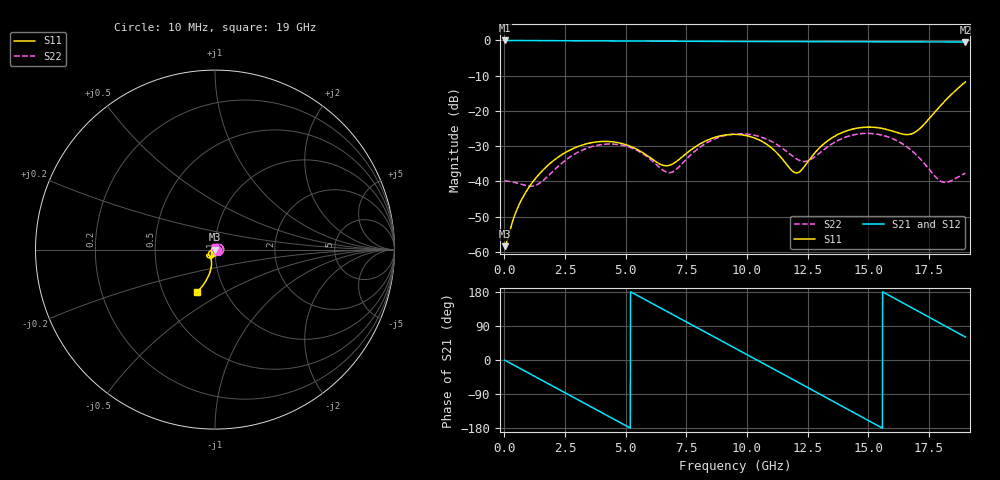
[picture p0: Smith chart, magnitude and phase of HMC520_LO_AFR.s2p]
! Analog Devices, Inc.
! 1 Analog Way
! Wilmington, MA 01887
! http://www.analog.com
! Date:  2021-09-07 NN
! Board Name:  EV1HMC520ALC4 Revision A with HMC520ALC4 installed
! File Description:  Automatic Fixture Removal S-Parameters for LO Port connector and board loss de-embedding
! File Generation:  Calibrated Network Analyzer
! Chip Part Number:  HMC520A
! Chip Description:  GaAs, MMIC, IQ Mixer
! Chip Frequency:  6 to 10 GHz
! Chip Package:  LCC, 3.9 x 3.9 x 0.9 mm
! LO Port:  HMC520ALC4 removed and end of trace left open
!Note:
!  Analog Devices supplies this data as a sample of measured data at the evaluation board
!  ports for this product.  Your particular data for this product may vary.
!  Analog Devices reserves the right to change this data at anytime.
!  All lines below in this file are as is from the Network Analyzer.
!Agilent Technologies,N5245A,MY52451809,A.10.47.06
!Automatic Fixture Removal (AFR)
!Date: Friday, August 27, 2021 11:21:52 PM
!S2P File: Measurements: S11,S21,S12,S22:
# MHz S  RI  R 50
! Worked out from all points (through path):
!   1900 points, 10 MHz to 19 GHz, reference 50 ohm
!   highest |S21| = 0.00 dB at 10 MHz (marker M1); lowest = -0.4 dB at 19 GHz (marker M2)
!   group delay of S21, straight-line fit = 96.3 ps
!   lowest |S11| = -58.4 dB at 10 MHz (marker M3), VSWR 1.00, Z = 50.1 + j0.0055 ohm
!   |S11| at or under -10 dB: start of sweep to end of sweep
!   |S22| runs from -41.4 to -26.4 dB; largest |S21 - S12| = 1.4e-15
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10  0.0012 5.49e-05  0.9999 -0.00602  0.9999 -0.00602  0.0101 2.59e-06
580  0.0037 0.00247  0.9371 -0.3413  0.9371 -0.3413  0.00931 0.000527
1200  0.0101 0.00102  0.7453 -0.6575  0.7453 -0.6575  0.008 0.00317
2210  0.0173 -0.0135  0.2332 -0.9608  0.2332 -0.9608  0.0119 0.0111
3180  0.00897 -0.0312  -0.3365 -0.9254  -0.3365 -0.9254  0.025 0.0114
4820  -0.0193 -0.0287  -0.9526 -0.2225  -0.9526 -0.2225  0.0278 -0.0172
5570  -0.0203 -0.0181  -0.9516 0.2167  -0.9516 0.2167  0.0108 -0.0239
6340  -0.0124 -0.0132  -0.7521 0.619  -0.7521 0.619  -0.0077 -0.0144
6920  -0.00574 -0.0166  -0.4938 0.8381  -0.4938 0.8381  -0.0135 0.00176
7900  -0.00496 -0.031  0.0561 0.9691  0.0561 0.9691  0.00212 0.0276
8670  -0.0161 -0.0389  0.4828 0.8403  0.4828 0.8403  0.0279 0.0286
9510  -0.031 -0.0345  0.8285 0.5  0.8285 0.5  0.0466 0.00599
10990  -0.0288 -0.00907  0.9067 -0.3325  0.9067 -0.3325  0.0162 -0.0334
12000  -0.00893 -0.00974  0.5497 -0.7923  0.5497 -0.7923  -0.016 -0.014
12670  -0.00158 -0.0224  0.1908 -0.9439  0.1908 -0.9439  -0.0168 0.0123
14030  -0.0201 -0.0469  -0.5628 -0.7771  -0.5628 -0.7771  0.0285 0.0308
14970  -0.0414 -0.0418  -0.8915 -0.3488  -0.8915 -0.3488  0.048 0.00128
15840  -0.0448 -0.0294  -0.9444 0.1488  -0.9444 0.1488  0.0331 -0.0264
16760  -0.0292 -0.0367  -0.7198 0.6276  -0.7198 0.6276  0.00302 -0.0276
17530  -0.0193 -0.077  -0.357 0.8845  -0.357 0.8845  -0.0102 -0.0103
18130  -0.0301 -0.1318  -0.0163 0.9527  -0.0163 0.9527  -0.00906 0.00336
19000  -0.1002 -0.2381  0.4676 0.8284  0.4676 0.8284  -0.00133 0.013
